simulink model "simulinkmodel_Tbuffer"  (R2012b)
settings: Solver=ode3  StartTime=0.0  StopTime=3600*24  FixedStep=60  RelTol=1e-12
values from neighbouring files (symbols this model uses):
  qinlb = qin_min    (= 0)    [objective_generall.m]
  qinub = qin_max    (= 10)    [objective_generall.m]
  Qlb = Qmin    (= 0)    [objective_generall.m]
  Qub = Qmax    (= 5.5)    [objective_generall.m]
libraries: simulink x2

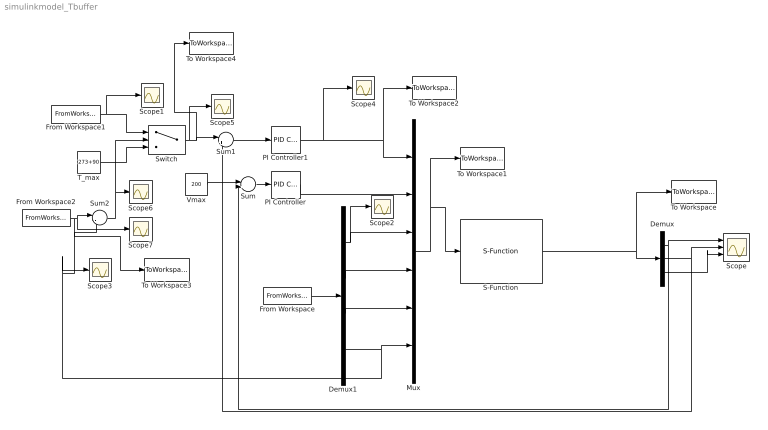
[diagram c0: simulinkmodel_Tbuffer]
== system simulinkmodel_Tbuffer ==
  Demux : Demux  Outputs=3
  Demux1 : Demux
  From Workspace : FromWorkspace  VariableName=dsim  SampleTime=0  OutputAfterFinalValue=Setting to zero
  From Workspace1 : FromWorkspace  VariableName=Tbuffer  SampleTime=0  Interpolate=off  OutputAfterFinalValue=Holding final value
  From Workspace2 : FromWorkspace  VariableName=Pthreshold  SampleTime=0  Interpolate=off  OutputAfterFinalValue=Holding final value
  Mux : Mux  Inputs=6
  PI Controller : simulink/Continuous/PID Controller  Controller=PI  TimeDomain=Continuous-time  SampleTime=1  IntegratorMethod=Forward Euler  FilterMethod=Forward Euler  Form=Ideal  P=3  I=1/80  D=0  N=100  InitialConditionSource=internal  InitialConditionForIntegrator=0  InitialConditionForFilter=0  ExternalReset=none  LimitOutput=on  UpperSaturationLimit=qinub  LowerSaturationLimit=qinlb  LinearizeAsGain=on  AntiWindupMode=clamping  Kb=1  TrackingMode=off  Kt=1  PParamMin=[]  PParamMax=[]  IParamMin=[]  IParamMax=[]  DParamMin=[]  DParamMax=[]  NParamMin=[]  NParamMax=[]  KbParamMin=[]  KbParamMax=[]  KtParamMin=[]  KtParamMax=[]  POutMin=[]  POutMax=[]  IOutMin=[]  IOutMax=[]  DOutMin=[]  DOutMax=[]  NOutMin=[]  NOutMax=[]  KbOutMin=[]  KbOutMax=[]  KtOutMin=[]  KtOutMax=[]  IntegratorOutMin=[]  IntegratorOutMax=[]  FilterOutMin=[]  FilterOutMax=[]  SumOutMin=[]  SumOutMax=[]  SumI1OutMin=[]  SumI1OutMax=[]  SumI2OutMin=[]  SumI2OutMax=[]  SumI3OutMin=[]  SumI3OutMax=[]  SumDOutMin=[]  SumDOutMax=[]  SaturationOutMin=[]  SaturationOutMax=[]  IntegratorContinuousStateAttributes=''  IntegratorStateMustResolveToSignalObject=off  IntegratorRTWStateStorageClass=Auto  FilterContinuousStateAttributes=''  FilterStateMustResolveToSignalObject=off  FilterRTWStateStorageClass=Auto
  PI Controller1 : simulink/Continuous/PID Controller  Controller=PI  TimeDomain=Continuous-time  SampleTime=1  IntegratorMethod=Forward Euler  FilterMethod=Forward Euler  Form=Ideal  P=50  I=1/80  D=0  N=100  InitialConditionSource=internal  InitialConditionForIntegrator=0  InitialConditionForFilter=0  ExternalReset=none  LimitOutput=on  UpperSaturationLimit=Qub  LowerSaturationLimit=Qlb  LinearizeAsGain=on  AntiWindupMode=clamping  Kb=1  TrackingMode=off  Kt=1  PParamMin=[]  PParamMax=[]  IParamMin=[]  IParamMax=[]  DParamMin=[]  DParamMax=[]  NParamMin=[]  NParamMax=[]  KbParamMin=[]  KbParamMax=[]  KtParamMin=[]  KtParamMax=[]  POutMin=[]  POutMax=[]  IOutMin=[]  IOutMax=[]  DOutMin=[]  DOutMax=[]  NOutMin=[]  NOutMax=[]  KbOutMin=[]  KbOutMax=[]  KtOutMin=[]  KtOutMax=[]  IntegratorOutMin=[]  IntegratorOutMax=[]  FilterOutMin=[]  FilterOutMax=[]  SumOutMin=[]  SumOutMax=[]  SumI1OutMin=[]  SumI1OutMax=[]  SumI2OutMin=[]  SumI2OutMax=[]  SumI3OutMin=[]  SumI3OutMax=[]  SumDOutMin=[]  SumDOutMax=[]  SaturationOutMin=[]  SaturationOutMax=[]  IntegratorContinuousStateAttributes=''  IntegratorStateMustResolveToSignalObject=off  IntegratorRTWStateStorageClass=Auto  FilterContinuousStateAttributes=''  FilterStateMustResolveToSignalObject=off  FilterRTWStateStorageClass=Auto
  S-Function : S-Function  FunctionName=sfunctionmodel  Parameters=par  EnableBusSupport=off
  Scope : Scope  NumInputPorts=3
  Scope{1..7} (7 alike) : Scope
  Sum : Sum  Inputs=|+-
  Sum1 : Sum  Inputs=|+-
  Sum2 : Sum  Inputs=|-+
  Switch : Switch
  T_max : Constant  Value=273+90
  To Workspace : ToWorkspace  VariableName=simout  SampleTime=-1  SaveFormat=Structure With Time
  To Workspace1 : ToWorkspace  VariableName=u  SampleTime=-1  SaveFormat=Structure With Time
  To Workspace2 : ToWorkspace  VariableName=simout1  SampleTime=-1  SaveFormat=Structure With Time
  To Workspace3 : ToWorkspace  VariableName=simout2  SampleTime=-1  SaveFormat=Structure With Time
  To Workspace4 : ToWorkspace  VariableName=simout3  SampleTime=-1  SaveFormat=Structure With Time
  Vmax : Constant  Value=200
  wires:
  Mux/1 -> To Workspace1/1, S-Function/1
  Demux/1 -> Sum/2, Scope/1
  Demux/2 -> Scope/2, Sum1/2
  Vmax/1 -> Sum/1
  Sum/1 -> PI Controller/1
  PI Controller/1 -> Mux/2
  S-Function/1 -> To Workspace/1, Demux/1
  Sum1/1 -> PI Controller1/1
  PI Controller1/1 -> Scope4/1, To Workspace2/1, Mux/1
  From Workspace/1 -> Demux1/1
  Demux1/1 -> Scope2/1, Mux/3
  Demux1/2 -> Mux/4
  Demux1/3 -> Mux/5
  Demux1/4 -> Sum2/2, Scope3/1, Mux/6
  Demux/3 -> Scope/3
  Switch/1 -> Scope5/1, To Workspace4/1, Sum1/1
  T_max/1 -> Switch/3
  From Workspace1/1 -> Scope1/1, Switch/1
  From Workspace2/1 -> To Workspace3/1, Scope7/1, Sum2/1
  Sum2/1 -> Scope6/1, Switch/2
